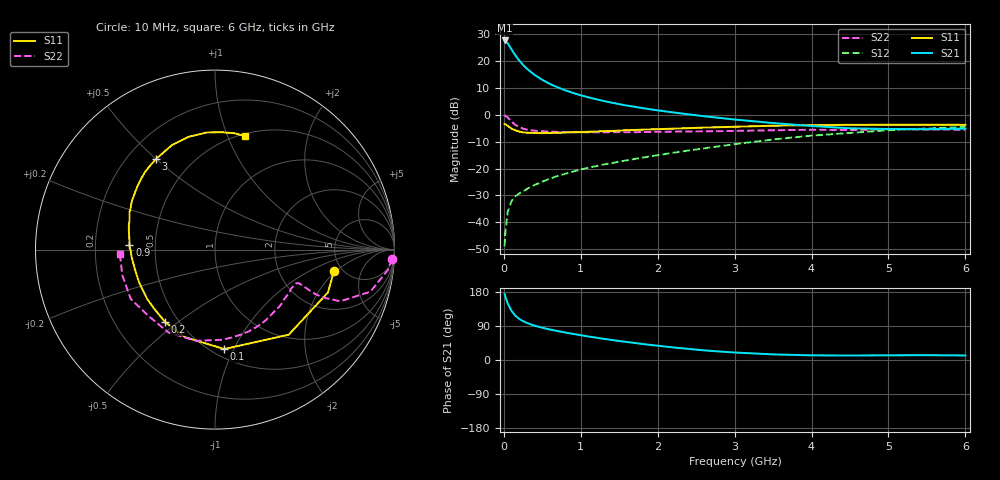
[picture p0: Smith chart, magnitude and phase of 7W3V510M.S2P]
! Infineon Technologies  Discrete & RF Semiconductors
! BFS17W
! Si NPN RF Bipolar Junction Transistor in SOT323
! VCE = 3.5 V  IC = 10 mA
! Common Emitter S-Parameters:  August  1999
# GHz  S  MA  R  50
!  f  S11  S21  S12  S22
! GHz  MAG  ANG  MAG  ANG  MAG  ANG  MAG  ANG
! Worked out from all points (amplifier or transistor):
!   36 points, 10 MHz to 6 GHz, reference 50 ohm
!   highest |S21| = 27.7 dB at 10 MHz (marker M1)
!   |S21| within 3 dB of that: start of sweep to 92.92 MHz
!   unconditionally stable (mu >= 1): 399.6 MHz to 2.474 GHz; 4.559 GHz to end of sweep
!   at 250 MHz: K = 0.80, MSG = 23.5 dB, |S12| = -28.4 dB
!   at 1.4 GHz: K = 1.21, MAG = 8.5 dB, |S12| = -18.0 dB
!   at 6 GHz: K = 1.07, MAG = -1.9 dB, |S12| = -4.5 dB
!   S11 on the Smith chart (normalised r, x): 10 MHz: 4.24, -1.89; 100 MHz: 0.57, -0.92; 200 MHz: 0.42, -0.45; 900 MHz: 0.35, +0.02; 3 GHz: 0.32, +0.50; 6 GHz: 0.52, +1.15
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0.01  0.6732 -10.4  24.38 173.8  0.0036 81.9  0.9871 -3.0
0.02  0.6732 -20.8  23.98 167.0  0.0065 79.3  0.9692 -6.8
0.05  0.6273 -49.1  21.6 149.7  0.0155 71.5  0.8963 -15.2
0.1  0.5563 -84.7  16.64 129.6  0.025 58.5  0.7552 -22.4
0.15  0.5157 -108.8  12.88 116.7  0.0305 53.4  0.6531 -24.0
0.2  0.49 -124.4  10.33 108.5  0.0345 53.2  0.5954 -23.8
0.25  0.4727 -135.6  8.538 102.5  0.0379 53.9  0.5572 -23.0
0.3  0.4674 -143.8  7.252 97.8  0.0418 55.3  0.5355 -22.5
0.4  0.461 -156.0  5.565 90.6  0.0497 57.6  0.5078 -21.9
0.5  0.4589 -164.0  4.501 85.2  0.0573 59.7  0.4965 -22.1
0.6  0.4611 -169.8  3.77 80.4  0.0652 62.0  0.4881 -22.8
0.7  0.4662 -174.8  3.263 76.3  0.0732 63.5  0.4835 -24.2
0.9  0.4774 177.1  2.566 68.9  0.088 64.9  0.4765 -27.6
1.1  0.4863 170.0  2.125 62.0  0.1041 66.1  0.4762 -31.9
1.3  0.4995 163.8  1.818 55.8  0.1198 66.8  0.4746 -36.7
1.6  0.5208 156.0  1.495 47.4  0.143 67.5  0.477 -44.2
2.2  0.5555 141.6  1.115 33.2  0.1972 68.5  0.4891 -61.3
3  0.6025 123.0  0.822 19.8  0.2854 65.4  0.504 -85.6
3.5  0.6297 112.4  0.706 14.8  0.3492 61.3  0.5188 -101.7
4.5  0.6542 93.9  0.564 11.8  0.4626 48.9  0.5235 -135.2
5.5  0.6573 80.6  0.542 12.7  0.56 36.2  0.5359 -164.5
6  0.6542 75.4  0.556 12.0  0.5977 30.1  0.5303 -177.3
